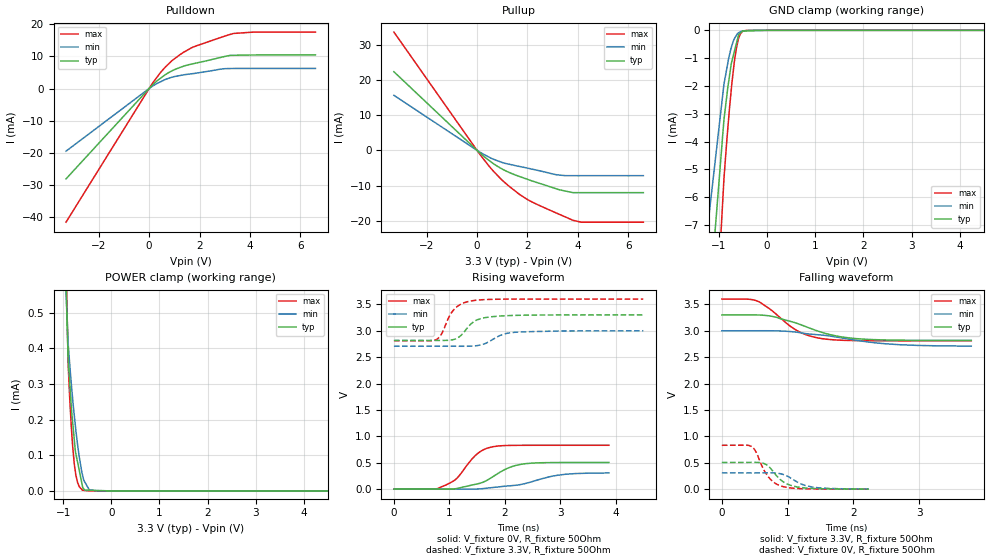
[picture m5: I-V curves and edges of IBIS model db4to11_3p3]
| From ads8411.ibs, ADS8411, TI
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|   db4to11_3p3 Model
[Model]   db4to11_3p3
Model_type   3-state
Polarity   Non-Inverting
Vmeas = 1.65
Vref = 1.65
Cref = 20pF
Rref = 50
|   typ   min   max
|   (nom PVT)   (fast PVT)   (slow PVT)
|C_comp from frequency sweep method (F=1MHz)
|C_comp   3.373e-12   3.314e-12   3.433e-12
|ON state : BUFFER OUTPUT TURNED HIGH
|C_comp   3.373e-12   3.314e-12   3.433e-12
|OFF state: BUFFER IN HIGH IMPEDANCE
|C_comp   3.339e-12   3.286e-12   3.396e-12
|C_comp from LC tank measurement(L=1nH)
|Resonant Frequency(Hz)   3.050e+09   3.080e+09   3.010e+09
C_comp   2.726e-12   2.673e-12   2.799e-12
|ON state : BUFFER OUTPUT TURNED HIGH
|Resonant Frequency(Hz)   3.050e+09   3.080e+09   3.020e+09
|C_comp   2.726e-12   2.673e-12   2.780e-12
|OFF state: BUFFER IN HIGH IMPEDANCE
|Resonant Frequency(Hz)   3.050e+09   3.080e+09   3.010e+09
|C_comp   2.726e-12   2.673e-12   2.799e-12
| Where nom  PVT is Nominal Process, 3.3V, 40C
|   Fast PVT is Strong Process,  3.6V, -40C
|   Slow PVT is Weak Process,   3V, 100C
[Voltage Range]   3.3   3   3.6
|Ambient Temperature   25   85   -40
|Junction Temperature
[Temperature Range]   40   100   -40
[Pullup Reference]   3.3   3   3.6
[Pulldown Reference]   0   0   0
[Power Clamp Reference]   3.3   3   3.6
[GND Clamp Reference]   0   0   0
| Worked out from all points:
|   slope of the pulldown table from 0 to 0.495 V, typ, clamps not added: 143 ohm
|   slope of the pullup table from 0 to 0.495 V, typ, clamps not added: 168 ohm
|   GND clamp passes 1 mA (typ) near -0.72 V on its own axis
|   falling waveform, V_fixture 3.3V, R_fixture 50Ohm: 20-80 % time 726ps typ, 1.07ns min, 503ps max; typ from 3.3 V to 2.82 V
|   rising waveform, V_fixture 0V, R_fixture 50Ohm: 20-80 % time 561ps typ, 795ps min, 410ps max; typ from 0 V to 0.505 V
|   rising waveform, V_fixture 3.3V, R_fixture 50Ohm: 20-80 % time 283ps typ, 343ps min, 248ps max; typ from 2.82 V to 3.3 V
|   falling waveform, V_fixture 0V, R_fixture 50Ohm: 20-80 % time 256ps typ, 293ps min, 221ps max; typ from 0.505 V to 0.001 V
[Pulldown]
|   Voltage   I(typ)   I(min)   I(max)
-3.3V     -28.14mA   -19.51mA   -41.61mA
126mV     1.005mA    697.4uA    1.535mA
478.8mV   3.358mA    2.196mA    5.234mA
939.6mV   5.626mA    3.599mA    8.872mA
1.372V    6.953mA    4.268mA    11.31mA
1.706V    7.639mA    4.605mA    12.76mA
2.934V    9.846mA    6.13mA     16.14mA
3.344V    10.34mA    6.23mA     17.13mA
4.162V    10.44mA    6.251mA    17.56mA
6.6V      10.48mA    6.251mA    17.56mA
[GND Clamp]
|   Voltage   I(typ)   I(min)   I(max)
-3.3V     -645.3mA   -463.1mA   -985.5mA
-1.541V   -17.22mA   -11.71mA   -25.7mA
-897.6mV  -3.221mA   -1.945mA   -5.352mA
-835.2mV  -2.32mA    -1.35mA    -3.909mA
-745.8mV  -1.202mA   -627.7uA   -2.153mA
-730.8mV  -1.1mA     -542.8uA   -1.883mA
-684mV    -782.4uA   -309.7uA   -1.175mA
-640.8mV  -489.3uA   -187.5uA   -665.9uA
-590.7mV  -149.4uA   -84.12uA   -284.5uA
-558mV    -100.4uA   -50.96uA   -133.3uA
-360mV    -18.26uA   -912.9nA   -156.2nA
6.6V      0A         0A         0A
[Pullup]
|   Voltage   I(typ)   I(min)   I(max)
-3.3V     22.37mA    15.66mA    33.65mA
172.8mV   -1.117mA   -764.9uA   -1.711mA
543.6mV   -3.215mA   -2.181mA   -5.053mA
939.6mV   -5.084mA   -3.294mA   -8.094mA
1.649V    -7.339mA   -4.529mA   -12.33mA
2.167V    -8.656mA   -5.311mA   -14.62mA
3.241V    -11.16mA   -7.006mA   -18.11mA
3.802V    -12.02mA   -7.192mA   -19.88mA
4.133V    -12.02mA   -7.192mA   -20.43mA
6.6V      -12.02mA   -7.192mA   -20.43mA
[POWER Clamp]
|   Voltage   I(typ)   I(min)   I(max)
-3.3V     638.7mA    457.7mA    976.4mA
-1.523V   3.32mA     2.55mA     4.556mA
-897.6mV  375.3uA    417.9uA    364.2uA
-864mV    305.6uA    355.7uA    261uA
-831.6mV  238.4uA    301.9uA    181.9uA
-770.4mV  146.2uA    214.1uA    78.28uA
-745.8mV  110.5uA    182.3uA    53.42uA
-702mV    81.49uA    131.6uA    24.44uA
-601.2mV  14.79uA    46.65uA    2.01uA
-459mV    2.105uA    3.326uA    248.6nA
-285mV    1.301uA    42.46nA    0A
6.6V      0A         0A         0A
[Ramp]
R_load = 50
|   typ   min   max
dV/dt_r   0.303293/5.60028e-10   0.184724/7.93751e-10   0.498804/4.08175e-10
dV/dt_f   0.289436/7.26265e-10   0.175537/1.0715e-09   0.474127/5.03055e-10
[Falling Waveform]
V_fixture = 3.3V
V_fixture_min = 3V
V_fixture_max = 3.6V
R_fixture = 50Ohm
|   Time   V(typ)   V(min)   V(max)
0s        3.3V       3V         3.6V
405ps     3.3V       3V         3.598V
548ps     3.299V     3V         3.558V
803ps     3.263V     2.999V     3.339V
1.137ns   3.142V     2.973V     3.008V
1.518ns   2.97V      2.919V     2.852V
1.809ns   2.886V     2.868V     2.821V
2.169ns   2.84V      2.796V     2.812V
2.707ns   2.822V     2.736V     2.81V
3.792ns   2.818V     2.709V     2.81V
[Rising Waveform]
V_fixture = 0V
V_fixture_min = 0V
V_fixture_max = 0V
R_fixture = 50Ohm
|   Time   V(typ)   V(min)   V(max)
0s        1.364nV    2.286nV    1.294nV
812ps     -64.35uV   -10.35uV   21.47mV
1.124ns   10.52mV    -45.53uV   194.6mV
1.404ns   77.46mV    612.2uV    567.4mV
1.524ns   104.6mV    3.889mV    686.4mV
1.795ns   242.9mV    32.92mV    805.6mV
2.057ns   399mV      61.03mV    827.5mV
2.39ns    484.3mV    112mV      830.8mV
3.095ns   504.7mV    282.1mV    831.3mV
3.877ns   505.4mV    306.8mV    831.3mV
[Rising Waveform]
V_fixture = 3.3V
V_fixture_min = 3V
V_fixture_max = 3.6V
R_fixture = 50Ohm
|   Time   V(typ)   V(min)   V(max)
0s        2.818V     2.707V     2.81V
772ps     2.817V     2.707V     2.836V
865ps     2.817V     2.707V     2.949V
1.08ns    2.835V     2.707V     3.398V
1.211ns   2.913V     2.706V     3.505V
1.385ns   3.124V     2.708V     3.563V
1.618ns   3.243V     2.747V     3.589V
1.961ns   3.281V     2.929V     3.598V
2.178ns   3.291V     2.971V     3.599V
4.499ns   3.3V       3V         3.6V
[Falling Waveform]
V_fixture = 0V
V_fixture_min = 0V
V_fixture_max = 0V
R_fixture = 50Ohm
|   Time   V(typ)   V(min)   V(max)
0s        505.5mV    308.1mV    831.3mV
452ps     507.3mV    308.1mV    806.8mV
514ps     507.3mV    308.3mV    716.7mV
625ps     492mV      309.3mV    397.4mV
693ps     449.4mV    309.8mV    256.3mV
788ps     321.5mV    307.7mV    132mV
918ps     152.7mV    283.7mV    52.93mV
1.095ns   55.23mV    172.5mV    17.34mV
1.366ns   14.74mV    42.47mV    3.799mV
2.234ns   708.8uV    2.752mV    76.25uV
